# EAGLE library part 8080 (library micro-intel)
MICROCOMPUTER/PERIPHERAL DEVICE
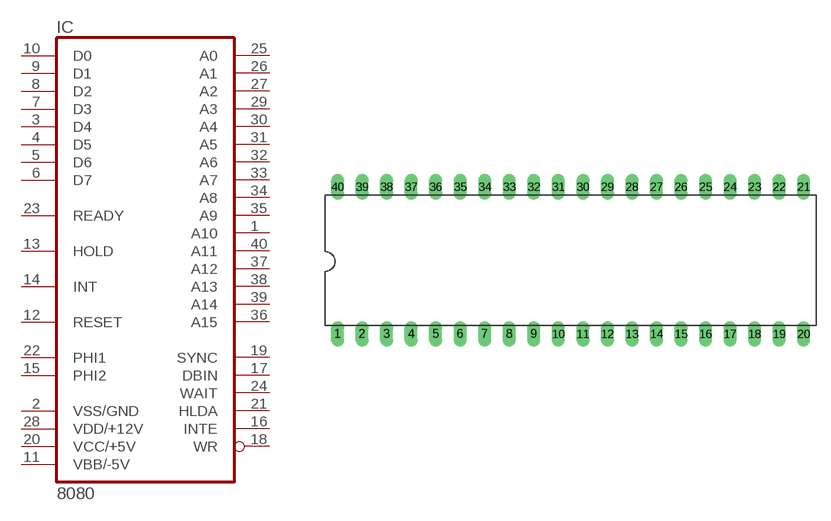
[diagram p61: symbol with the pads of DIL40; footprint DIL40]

Designator prefix IC

## 8080 (OC_FARNELL: unknown; OC_NEWARK: unknown)  [DIL40]
1  A10  out
2  VSS/GND  pwr
3  D4
4  D5
5  D6
6  D7
7  D3
8  D2
9  D1
10  D0
11  VBB/-5V  pwr
12  RESET  in
13  HOLD  in
14  INT  in
15  PHI2  in
16  INTE  out
17  DBIN  out
18  WR  out
19  SYNC  out
20  VCC/+5V  pwr
21  HLDA  out
22  PHI1  in
23  READY  in
24  WAIT  out
25  A0  out
26  A1  out
27  A2  out
28  VDD/+12V  pwr
29  A3  out
30  A4  out
31  A5  out
32  A6  out
33  A7  out
34  A8  out
35  A9  out
36  A15  out
37  A12  out
38  A13  out
39  A14  out
40  A11  out

## Footprint DIL40 (pad centres in mm)
Dual In Line Package
drill 0.813 long: 1 -24.13,-7.62; 2 -21.59,-7.62; 3 -19.05,-7.62; 4 -16.51,-7.62; 5 -13.97,-7.62; 6 -11.43,-7.62; 7 -8.89,-7.62; 8 -6.35,-7.62; 9 -3.81,-7.62; 10 -1.27,-7.62; 11 1.27,-7.62; 12 3.81,-7.62; 13 6.35,-7.62; 14 8.89,-7.62; 15 11.43,-7.62; 16 13.97,-7.62; 17 16.51,-7.62; 18 19.05,-7.62; 19 21.59,-7.62; 20 24.13,-7.62; 21 24.13,7.62; 22 21.59,7.62; 23 19.05,7.62; 24 16.51,7.62; 25 13.97,7.62; 26 11.43,7.62; 27 8.89,7.62; 28 6.35,7.62; 29 3.81,7.62; 30 1.27,7.62; 31 -1.27,7.62; 32 -3.81,7.62; 33 -6.35,7.62; 34 -8.89,7.62; 35 -11.43,7.62; 36 -13.97,7.62; 37 -16.51,7.62; 38 -19.05,7.62; 39 -21.59,7.62; 40 -24.13,7.62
